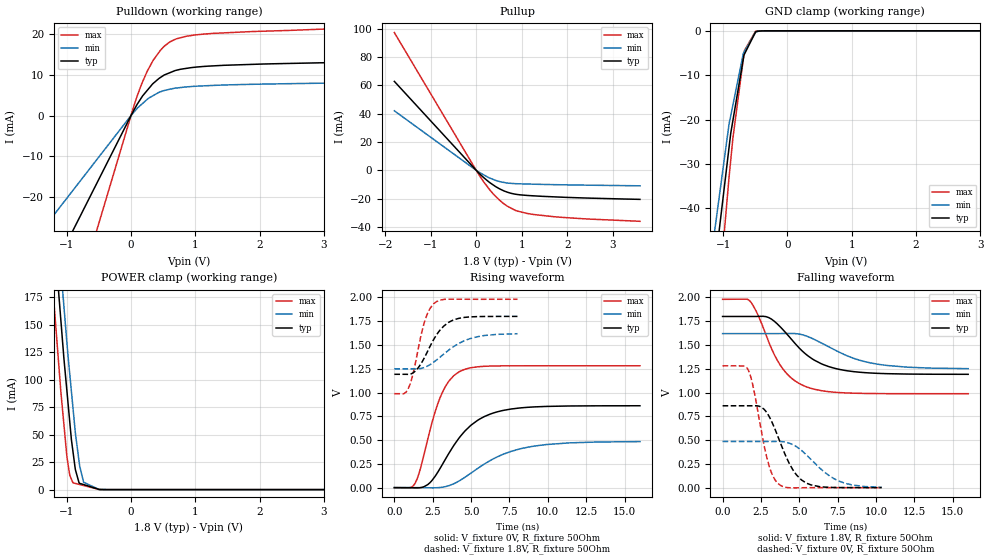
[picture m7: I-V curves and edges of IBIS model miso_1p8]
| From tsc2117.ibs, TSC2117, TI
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|   miso_1p8 Model
[Model]   miso_1p8
Model_type   3-state
Polarity   Non-Inverting
Vmeas = 0.9
Vref = 0.9
Cref = 10pF
Rref = 50
|   typ   min   max
|   (nom PVT)   (fast PVT)   (slow PVT)
|C_comp from frequency sweep method (F=25MHz)
|C_comp   4.313e-12   4.005e-12   4.366e-12
|ON state : BUFFER OUTPUT TURNED HIGH
|C_comp   4.313e-12   4.005e-12   4.366e-12
|OFF state: BUFFER IN HIGH IMPEDANCE
|C_comp   1.687e-12   1.683e-12   1.689e-12
|C_comp from LC tank measurement(L=1nH)
|Resonant Frequency(Hz)   4.070e+09   4.140e+09   4.020e+09
C_comp   1.531e-12   1.479e-12   1.569e-12
|ON state : BUFFER OUTPUT TURNED HIGH
|Resonant Frequency(Hz)   4.070e+09   4.140e+09   4.020e+09
|C_comp   1.531e-12   1.479e-12   1.569e-12
|OFF state: BUFFER IN HIGH IMPEDANCE
|Resonant Frequency(Hz)   4.250e+09   4.280e+09   4.247e+09
|C_comp   1.404e-12   1.384e-12   1.405e-12
| Where nom  PVT is Nominal Process, 1.8V, 48C
|   Fast PVT is Strong Process,  1.98V, -40C
|   Slow PVT is Weak Process,   1.62V, 108C
[Voltage Range]   1.8   1.62   1.98
|Ambient Temperature   25   85   -40
|Junction Temperature
[Temperature Range]   48   108   -40
[Pullup Reference]   1.8   1.62   1.98
[Pulldown Reference]   0   0   0
[Power Clamp Reference]   1.8   1.62   1.98
[GND Clamp Reference]   0   0   0
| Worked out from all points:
|   slope of the pulldown table from 0 to 0.27 V, typ, clamps not added: 41.3 ohm
|   slope of the pullup table from 0 to 0.27 V, typ, clamps not added: 34 ohm
|   GND clamp passes 1 mA (typ) near -0.52 V on its own axis
|   POWER clamp passes 1 mA (typ) near -0.54 V on its own axis
|   falling waveform, V_fixture 1.8V, R_fixture 50Ohm: 20-80 % time 2.48ns typ, 3.15ns min, 1.86ns max; typ from 1.8 V to 1.19 V
|   rising waveform, V_fixture 0V, R_fixture 50Ohm: 20-80 % time 2.4ns typ, 3.26ns min, 1.41ns max; typ from 0 V to 0.861 V
|   rising waveform, V_fixture 1.8V, R_fixture 50Ohm: 20-80 % time 1.33ns typ, 1.97ns min, 842ps max; typ from 1.19 V to 1.8 V
|   falling waveform, V_fixture 0V, R_fixture 50Ohm: 20-80 % time 1.43ns typ, 2.05ns min, 946ps max; typ from 0.861 V to 0 V
[Pulldown]
|   Voltage   I(typ)   I(min)   I(max)
-1.8V     -56.49mA   -36.75mA   -95.55mA
-72mV     -2.259mA   -1.47mA    -3.822mA
95.04mV   2.758mA    1.751mA    4.798mA
168.3mV   4.552mA    2.822mA    7.911mA
251.5mV   6.192mA    3.988mA    10.89mA
348.5mV   7.968mA    4.952mA    13.71mA
463.3mV   9.448mA    5.897mA    16.21mA
601.9mV   10.55mA    6.481mA    18.13mA
698.9mV   11.15mA    6.779mA    18.88mA
855.4mV   11.62mA    7.059mA    19.53mA
1.277V    12.25mA    7.427mA    20.26mA
3.6V      13.28mA    8.129mA    21.69mA
[GND Clamp]
|   Voltage   I(typ)   I(min)   I(max)
-1.8V     -204.2mA   -122.7mA   -346.2mA
-1.168V   -57.98mA   -48.96mA   -76.54mA
-910.4mV  -26.53mA   -21.21mA   -33.32mA
-882mV    -23.09mA   -19.13mA   -29.11mA
-847.4mV  -20.13mA   -16.65mA   -24.05mA
-686.9mV  -6.336mA   -5.106mA   -6.397mA
-676.8mV  -5.471mA   -4.853mA   -5.288mA
-669.2mV  -5.253mA   -4.663mA   -4.457mA
-495mV    -233.2uA   -288.5uA   -64.76uA
-309.4mV  -2uA       -3.404uA   -88.21nA
3.6V      0A         0A         0A
[Pullup]
|   Voltage   I(typ)   I(min)   I(max)
-1.8V     62.74mA    41.98mA    97.18mA
95.04mV   -3.093mA   -1.942mA   -4.857mA
348.5mV   -9.775mA   -6.119mA   -15.69mA
601.9mV   -14.42mA   -8.513mA   -23.45mA
683.1mV   -15.42mA   -8.991mA   -25.3mA
900.9mV   -17.04mA   -9.476mA   -28.73mA
1.277V    -18.04mA   -9.812mA   -31.23mA
2.376V    -19.52mA   -10.46mA   -34.22mA
3.6V      -20.5mA    -10.94mA   -35.98mA
[POWER Clamp]
|   Voltage   I(typ)   I(min)   I(max)
-1.8V     711.3mA    747.3mA    662mA
-1.215V   245.7mA    292.3mA    183mA
-1.129V   182.6mA    228.3mA    118.2mA
-1.044V   120mA      167.5mA    59.76mA
-994mV    88.16mA    131.9mA    28.81mA
-952.4mV  61.74mA    105.3mA    13.13mA
-902.9mV  34.89mA    74.83mA    6.212mA
-865.8mV  18.41mA    52.09mA    5.654mA
-806.4mV  5.838mA    25.14mA    4.761mA
-737.1mV  4.574mA    6.658mA    3.718mA
-494.1mV  154.3uA    103.9uA    74.57uA
3.6V      0A         0A         0A
[Ramp]
R_load = 50
|   typ   min   max
dV/dt_r   0.516429/2.3854e-09   0.290342/3.24284e-09   0.768595/1.40957e-09
dV/dt_f   0.365028/2.45984e-09   0.221333/3.14379e-09   0.59544/1.85871e-09
[Falling Waveform]
V_fixture = 1.8V
V_fixture_min = 1.62V
V_fixture_max = 1.98V
R_fixture = 50Ohm
|   Time   V(typ)   V(min)   V(max)
0s        1.8V       1.62V      1.98V
1.777ns   1.8V       1.62V      1.963V
2.196ns   1.8V       1.62V      1.853V
3.006ns   1.788V     1.62V      1.533V
3.774ns   1.688V     1.62V      1.284V
4.53ns    1.552V     1.621V     1.146V
5.454ns   1.4V       1.594V     1.061V
7.225ns   1.258V     1.455V     1.004V
9.629ns   1.206V     1.312V     989.8mV
16ns      1.192V     1.251V     987.6mV
[Rising Waveform]
V_fixture = 0V
V_fixture_min = 0V
V_fixture_max = 0V
R_fixture = 50Ohm
|   Time   V(typ)   V(min)   V(max)
0s        2.069nV    8.463nV    579.5pV
1.363ns   -2.152mV   64.27uV    48.93mV
2.186ns   33mV       -1.576mV   516mV
2.979ns   202mV      1.422mV    944.7mV
3.574ns   366.2mV    21.6mV     1.124V
4.3ns     538.8mV    77.89mV    1.224V
5.563ns   721.1mV    216.5mV    1.272V
7.589ns   825.9mV    380.1mV    1.281V
9.888ns   853.6mV    452.7mV    1.281V
16ns      860.7mV    483.9mV    1.281V
[Rising Waveform]
V_fixture = 1.8V
V_fixture_min = 1.62V
V_fixture_max = 1.98V
R_fixture = 50Ohm
|   Time   V(typ)   V(min)   V(max)
0s        1.191V     1.249V     987.6mV
643ps     1.191V     1.249V     989.3mV
919ps     1.191V     1.249V     1.045V
1.21ns    1.206V     1.249V     1.19V
1.973ns   1.37V      1.264V     1.746V
2.613ns   1.571V     1.325V     1.94V
3.23ns    1.699V     1.405V     1.979V
4.181ns   1.779V     1.514V     1.981V
5.823ns   1.799V     1.598V     1.98V
8.022ns   1.8V       1.618V     1.98V
[Falling Waveform]
V_fixture = 0V
V_fixture_min = 0V
V_fixture_max = 0V
R_fixture = 50Ohm
|   Time   V(typ)   V(min)   V(max)
0s        860.8mV    485.3mV    1.281V
1.683ns   860.8mV    485.3mV    1.234V
1.981ns   860.9mV    485.3mV    1.069V
2.907ns   782.8mV    485.3mV    302.2mV
3.221ns   687.8mV    485.3mV    142.7mV
3.606ns   536.9mV    485.4mV    43.91mV
4.569ns   190.5mV    452.7mV    -2.334mV
5.483ns   46.19mV    341.2mV    -540.1uV
7.676ns   742.2uV    62.63mV    5.54uV
10.37ns   12.1uV     3.495mV    39.25nV
